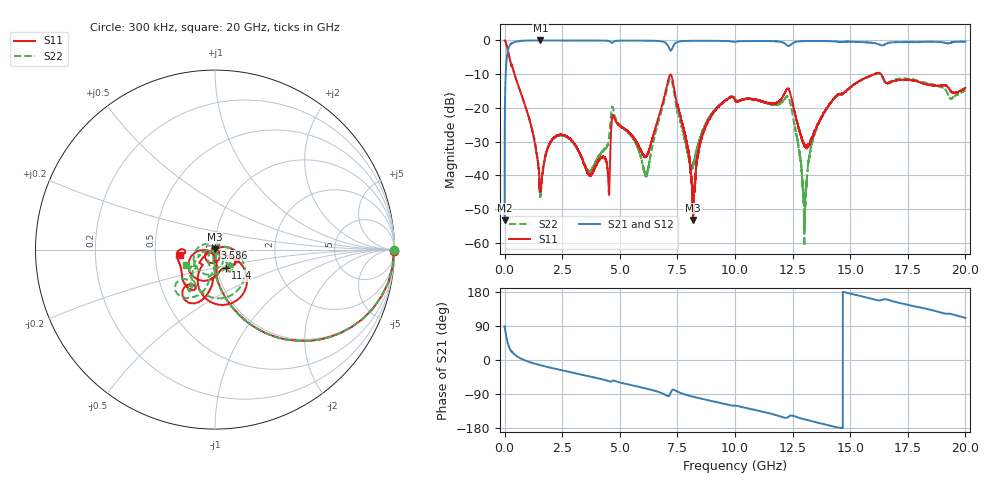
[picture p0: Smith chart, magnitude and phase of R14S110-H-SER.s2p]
!{R14S110}
!Johanson Technology Inc.
!www.johansontechnology.com
!Test Board Conditions:
!Substrate Type  RO4350B
!Substrate Thickness  20 mil
!Substrate Dk  3.66
!TL Type: GCPW
!TL Trace Width  36 mil
!TL Gap  12 mil
!Electrode orientation  Horizontal
!DUT TOPOLOGY	SERIES
!Mounting Pad LxW  26x36 mil
! Created Wed Nov 25 17:33:21 2020
! 2 Port Network Data from SP1.SP block
! freq  magS11  angS11  magS21  angS21  magS12  angS12  magS22  angS22
# khz S ma R 50
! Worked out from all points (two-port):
!   20001 points, 300 kHz to 20 GHz, reference 50 ohm
!   highest |S21| = 0.00 dB at 1.557 GHz (marker M1); lowest = -53.4 dB at 300 kHz (marker M2)
!   |S21| within 3 dB of the highest: 143.1 MHz to 7.196 GHz (7.053 GHz wide, 192 % of centre); 7.225 GHz to end of sweep
!   lowest |S11| = -53.3 dB at 8.178 GHz (marker M3), VSWR 1.00, Z = 49.9 + j0.198 ohm
!   |S11| at or under -10 dB: 428.6 MHz to 16.04 GHz (15.61 GHz wide, 190 % of centre); 16.34 GHz to end of sweep
!   |S22| runs from -61.1 to 0.0 dB; largest |S21 - S12| = 0.019
!   S11 on the Smith chart (normalised r, x): 300 kHz: open; 3.586 GHz: 1.00, +0.02; 11.4 GHz: 1.10, -0.23; 20 GHz: 0.67, -0.04
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300  0.9967 -0.3  0.002142 87.9  0.002116 90.0  0.9975 -0.3
103300  0.808 -36.9  0.5853 53.0  0.5871 53.0  0.8084 -36.8
195300  0.5827 -55.8  0.8089 33.9  0.8098 33.9  0.5841 -55.8
1557300  0.006023 -4.7  0.9998 -13.7  0.9987 -13.7  0.005124 162.1
2233300  0.03794 54.3  0.9978 -23.8  0.998 -23.8  0.03722 75.7
3334300  0.01863 59.6  0.9975 -38.7  0.9973 -38.7  0.01848 37.5
3586300  0.0112 87.0  0.9973 -42.0  0.9975 -42.0  0.01195 1.1
4489300  0.009917 138.2  0.9874 -55.1  0.987 -55.1  0.02986 -60.1
4707300  0.07887 -118.7  0.9444 -54.1  0.9451 -54.1  0.09906 -103.0
6143300  0.01916 -89.7  0.9924 -75.3  0.9925 -75.3  0.009608 114.8
6667300  0.0697 -26.1  0.983 -84.0  0.9816 -83.9  0.06055 15.4
7241300  0.3001 -91.1  0.7212 -82.1  0.721 -82.1  0.261 -99.5
8178300  0.002174 114.3  0.9891 -96.9  0.9887 -96.8  0.01393 -97.9
8786300  0.05846 14.3  0.9897 -105.5  0.9897 -105.5  0.06287 -51.3
1.00003e7  0.1294 -30.6  0.9526 -120.5  0.9518 -120.6  0.1378 -57.7
1.13973e7  0.1182 -59.3  0.98 -139.3  0.9784 -139.3  0.1163 -41.9
1.23503e7  0.1844 -140.7  0.8277 -148.5  0.8313 -148.6  0.1356 -149.7
1.30113e7  0.02706 -148.8  0.9787 -156.5  0.9778 -156.6  0.000885 32.6
1.33343e7  0.03595 -97.6  0.983 -161.7  0.9835 -161.6  0.02931 -81.4
1.44173e7  0.1516 -91.0  0.9613 -177.6  0.9627 -177.7  0.1495 -100.3
1.66673e7  0.2306 -119.0  0.9224 158.3  0.917 158.1  0.2356 -124.2
2e7  0.1983 -171.5  0.9591 111.0  0.9571 111.2  0.1825 -151.3
